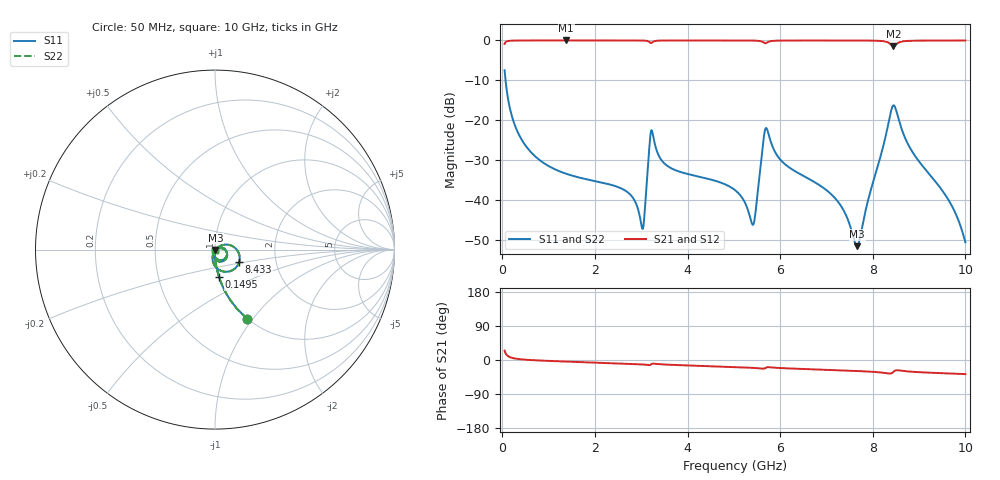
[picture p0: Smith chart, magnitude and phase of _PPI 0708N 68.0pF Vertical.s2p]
! S-Parameter data specifications (vertical orientation):
! Substrate: 40-mil Rogers 3003C, Substrate thickness, H=1.016mm, Dielectric constant, Er=3, Conductor thickness, T_mtl=0.043mm, Loss Tangent, Tand=0.003
! PCB Mounting Pad Footprint: Pad width, PadW=2.54mm , Pad length, PadL=0.51mm , Pad gap, PadG (edge-to-edge)=0.71mm , Reference planes=1.73mm apart
! Created Tue Jan 16 08:54:08 2018
# GHz S MA R 50
! 2 Port Network Data from SP1.SP block
! freq  magS11  angS11  magS21  angS21  magS12  angS12  magS22  angS22
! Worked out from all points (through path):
!   801 points, 50 MHz to 10 GHz, reference 50 ohm
!   highest |S21| = -0.01 dB at 1.381 GHz (marker M1); lowest = -1.5 dB at 8.445 GHz (marker M2)
!   group delay of S21, straight-line fit = 11.1 ps
!   lowest |S11| = -51.5 dB at 7.662 GHz (marker M3), VSWR 1.01, Z = 50.2 - j0.152 ohm
!   |S11| at or under -10 dB: 70.3 MHz to end of sweep
!   |S22| runs from -51.5 to -7.5 dB; largest |S21 - S12| = 0
!   S11 on the Smith chart (normalised r, x): 50 MHz: 1.00, -0.93; 149.5 MHz: 1.00, -0.31; 8.433 GHz: 1.30, -0.18; 10 GHz: 1.00, -0.01
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0.05  0.4232 -65.1  0.9058 24.8  0.9058 24.8  0.4232 -65.1
0.1495  0.1548 -81.6  0.9878 8.3  0.9878 8.3  0.1548 -81.6
0.5599375  0.0436 -89.3  0.9987 0.3  0.9987 0.3  0.0436 -89.3
1.380812  0.02138 -93.0  0.9993 -4.2  0.9993 -4.2  0.02138 -93.0
1.716625  0.01883 -94.1  0.9993 -5.6  0.9993 -5.6  0.01883 -94.1
2.68675  0.0128 -95.7  0.9989 -9.7  0.9989 -9.7  0.0128 -95.7
3.022562  0.004388 -44.3  0.9962 -11.6  0.9962 -11.6  0.004388 -44.3
3.209125  0.07234 -21.0  0.9284 -11.8  0.9284 -11.8  0.07234 -21.0
3.370812  0.0369 -91.7  0.9932 -11.0  0.9932 -11.0  0.0369 -91.7
5.025  0.01335 -102.3  0.9982 -18.6  0.9982 -18.6  0.01335 -102.3
5.423  0.004972 -34.0  0.9949 -20.8  0.9949 -20.8  0.004972 -34.0
5.634437  0.05338 0.4  0.9505 -22.9  0.9505 -22.9  0.05338 0.4
5.709062  0.07906 -53.8  0.9335 -19.4  0.9335 -19.4  0.07906 -53.8
6.02  0.03138 -104.1  0.9953 -21.3  0.9953 -21.3  0.03138 -104.1
6.691625  0.01749 -109.2  0.9979 -24.6  0.9979 -24.6  0.01749 -109.2
7.276187  0.009093 -105.6  0.9978 -27.2  0.9978 -27.2  0.009093 -105.6
7.66175  0.00265 -34.8  0.997 -29.1  0.997 -29.1  0.00265 -34.8
8.345812  0.09624 12.6  0.933 -35.7  0.933 -35.7  0.09624 12.6
8.432875  0.1516 -27.3  0.8486 -32.7  0.8486 -32.7  0.1516 -27.3
8.445312  0.1541 -35.0  0.8458 -31.3  0.8458 -31.3  0.1541 -35.0
8.793563  0.04626 -107.6  0.9883 -30.5  0.9883 -30.5  0.04626 -107.6
10  0.002959 -82.2  0.9975 -37.2  0.9975 -37.2  0.002959 -82.2
